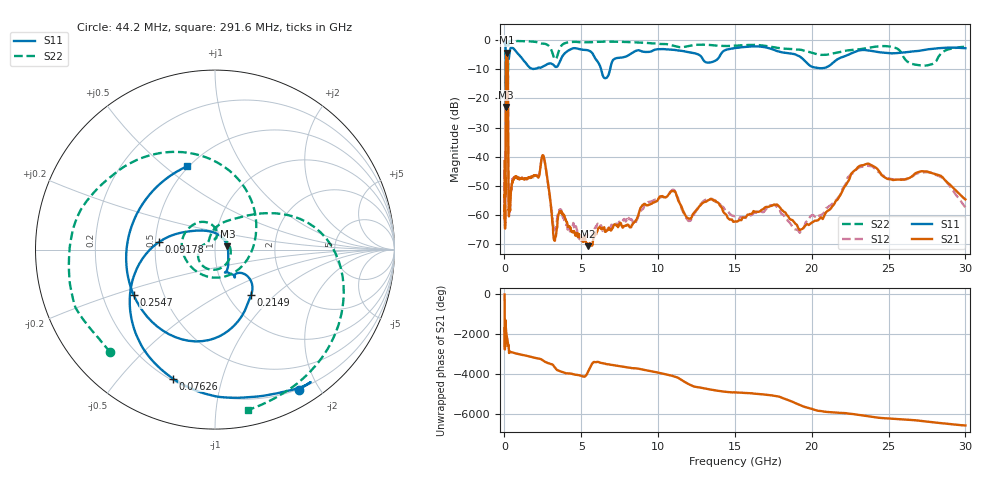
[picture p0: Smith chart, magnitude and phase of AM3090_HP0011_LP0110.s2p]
! Date/Time: Thu, Feb 28, 2019 1:56 PM
! Network Analyzer: Agilent Technologies E8364B Rev: A.07.50.67
! Sweep from 0.010 to 30.000 GHz, 1601 Points, Sweep Type: LOG
! Power Supply: 5.023 V, 0.002 A
# Hz S DB R 50
!freq MagS11 AngS11 MagS21 AngS21 MagS12 AngS12 MagS22 AngS22
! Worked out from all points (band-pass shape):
!   1601 points, 10 MHz to 30 GHz, reference 50 ohm
!   highest |S21| = -4.31 dB at 149.9 MHz (marker M1); lowest = -70.6 dB at 5.446 GHz (marker M2)
!   |S21| within 3 dB of the highest: 102.5 MHz to 210.6 MHz (108.1 MHz wide, 69 % of centre)
!   lowest |S11| = -23.0 dB at 100.4 MHz (marker M3), VSWR 1.15, Z = 57.3 + j2.14 ohm
!   |S11| at or under -10 dB: 91.77 MHz to 213.3 MHz (121.6 MHz wide, 79.7 % of centre); 6.288 GHz to 6.877 GHz (588.8 MHz wide, 8.95 % of centre)
!   |S22| runs from -24.9 to -0.2 dB; largest |S21 - S12| = 0.013
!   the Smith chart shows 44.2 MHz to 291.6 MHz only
!   S11 on the Smith chart (normalised r, x): 44.2 MHz: 0.19, -1.75; 76.26 MHz: 0.21, -0.70; 91.78 MHz: 0.52, +0.05; 214.9 MHz: 1.27, -0.72; 254.7 MHz: 0.34, -0.23; 291.6 MHz: 0.49, +0.60
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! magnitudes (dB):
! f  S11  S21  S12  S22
! 10 MHz  -0.3  -41.5  -44.3  -0.5
! 38.04 MHz  -0.5  -62.9  -61.5  -1.4
! 44.2 MHz  -0.8  -58.5  -58.3  -1.8
! 48.61 MHz  -0.8  -48.2  -50.6  -1.5
! 76.26 MHz  -2.4  -48.4  -49.4  -4.5
! 91.78 MHz  -10.0  -16.1  -16.1  -15.9
! 100.4 MHz  -23.0  -8.1  -8.1  -14.4
! 144.7 MHz  -15.5  -4.3  -4.3  -21.8
! 149.9 MHz  -15.3  -4.3  -4.3  -21.0
! 214.9 MHz  -9.8  -8.2  -8.2  -15.3
! 254.7 MHz  -5.7  -48.1  -48.3  -1.8
! 291.6 MHz  -6.2  -60.4  -58.2  -0.8
! 550.5 MHz  -2.8  -48.0  -47.7  -0.3
! 2.084 GHz  -9.8  -46.5  -46.3  -0.7
! 2.533 GHz  -9.0  -39.6  -39.8  -1.3
! 3.253 GHz  -9.0  -68.7  -65.1  -6.4
! 5.446 GHz  -3.6  -70.6  -67.1  -0.8
! 7.926 GHz  -5.6  -63.6  -61.9  -0.7
! 10.76 GHz  -3.3  -52.5  -52.3  -1.7
! 19.7 GHz  -8.0  -63.0  -61.9  -3.9
! 23.48 GHz  -3.5  -42.7  -43.2  -2.9
! 30 GHz  -2.8  -54.6  -57.3  -2.3
